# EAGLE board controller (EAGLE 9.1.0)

Size 100 x 80 mm. Coordinates in mm from the lower left corner, seen from the top.
Outline: 0,0 100,0 100,80 0,80 0,0
Copper layers (1*16): Top 0.035mm / dielectric 1.5mm / Bottom 0.035mm
Design rules "default": minimum track width 6mil, minimum drill 0.35mm, track to track 6mil, track to pad 6mil, pad to pad 6mil, via to via 6mil, smd to smd 6mil, copper to edge 40mil, drill to drill 6mil, minimum pad ring 10mil, minimum via ring 8mil, stop-mask expansion 4mil, vias tented up to drill 0mil, thermal gap 10mil

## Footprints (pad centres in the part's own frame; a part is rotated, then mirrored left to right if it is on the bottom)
ARDUINO_R3 = drill 1.016 pad 1.93: 3.3V 2.54,-24.13; 5V 5.08,-24.13; A0 17.78,-24.13; A1 20.32,-24.13; A2 22.86,-24.13; A3 25.4,-24.13; A4 27.94,-24.13; A5 30.48,-24.13; AREF -9.144,24.13; D0 30.48,24.13; D1 27.94,24.13; D2 25.4,24.13; D3 22.86,24.13; D4 20.32,24.13; D5 17.78,24.13; D6 15.24,24.13; D7 12.7,24.13; D8 8.636,24.13; D9 6.096,24.13; D10 3.556,24.13; D11 1.016,24.13; D12 -1.524,24.13; D13 -4.064,24.13; GND@1 7.62,-24.13; GND@2 10.16,-24.13; GND@3 -6.604,24.13; GND@4 33.16,-1.32; IOREF -2.54,-24.13; MISO 30.62,3.76; MOSI 33.16,1.22; NC -5.08,-24.13; RESET@1 0,-24.13; RESET@2 30.62,-1.32; SCK 30.62,1.22; SCL -14.224,24.13; SDA -11.684,24.13; VCC 33.16,3.76; VIN 12.7,-24.13 | hole 3.175: -17.78,24.13; 33.02,8.89; 33.02,-19.05; -19.05,-24.13
2X20_SHROUDED = drill 1.016 pad 1.88: 1 -1.27,24.13; 2 1.27,24.13; 3 -1.27,21.59; 4 1.27,21.59; 5 -1.27,19.05; 6 1.27,19.05; 7 -1.27,16.51; 8 1.27,16.51; 9 -1.27,13.97; 10 1.27,13.97; 11 -1.27,11.43; 12 1.27,11.43; 13 -1.27,8.89; 14 1.27,8.89; 15 -1.27,6.35; 16 1.27,6.35; 17 -1.27,3.81; 18 1.27,3.81; 19 -1.27,1.27; 20 1.27,1.27; 21 -1.27,-1.27; 22 1.27,-1.27; 23 -1.27,-3.81; 24 1.27,-3.81; 25 -1.27,-6.35; 26 1.27,-6.35; 27 -1.27,-8.89; 28 1.27,-8.89; 29 -1.27,-11.43; 30 1.27,-11.43; 31 -1.27,-13.97; 32 1.27,-13.97; 33 -1.27,-16.51; 34 1.27,-16.51; 35 -1.27,-19.05; 36 1.27,-19.05; 37 -1.27,-21.59; 38 1.27,-21.59; 39 -1.27,-24.13; 40 1.27,-24.13
1X03 = drill 1.016 pad 1.88: 1 0,0; 2 2.54,0; 3 5.08,0
0204/7 = drill 0.813 octagon: 1 -3.81,0; 2 3.81,0

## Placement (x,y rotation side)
B1  ARDUINO_UNO_R3  [ARDUINO_R3]  not placed on the board
J1  RASPBERRYPI-40-PIN-GPIO_PTH  [2X20_SHROUDED]  not placed on the board
M1  SERVO  [1X03]  not placed on the board
M2  SERVO  [1X03]  not placed on the board
M3  SERVO  [1X03]  not placed on the board
R1  22k  [0204/7]  not placed on the board
R2  1k  [0204/7]  not placed on the board

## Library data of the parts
B1 = SparkFun-Boards
J1 = SparkFun-Connectors; PROD_ID: CONN-12263; SF_ID: PRT-13054
M1-M3 = SparkFun-Electromechanical
R1 R2 = rcl; SPICEPREFIX: R

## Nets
3.3V: J1.1 J1.17
5V: J1.2 J1.4
GND: J1.6 J1.9 J1.14 J1.20 J1.25 J1.30 J1.34 J1.39

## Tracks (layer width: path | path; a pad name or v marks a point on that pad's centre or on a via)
3.3V  (1 unrouted)
5V  (1 unrouted)
GND  (7 unrouted)

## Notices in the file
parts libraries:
SparkFun-Boards: Licensing: Creative Commons ShareAlike 4.0 International - https://creativecommons.org/licenses/by-sa/4.0
